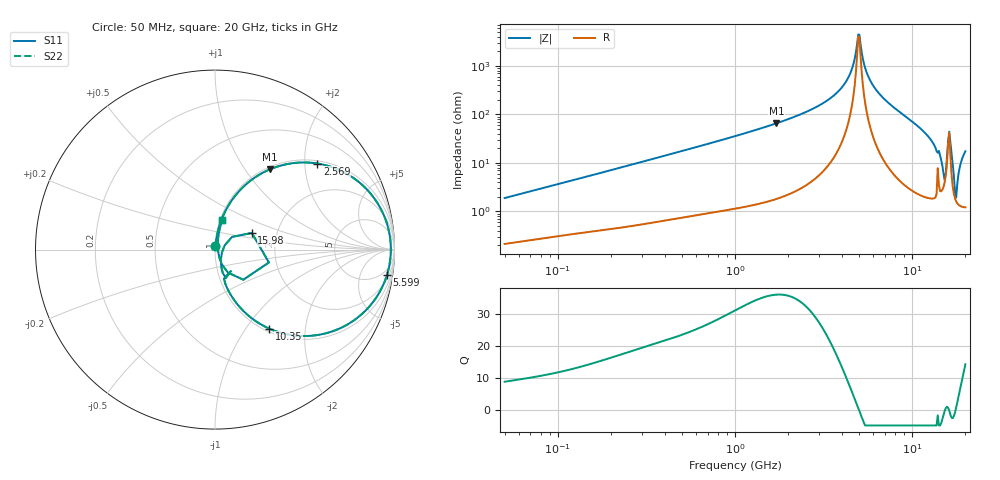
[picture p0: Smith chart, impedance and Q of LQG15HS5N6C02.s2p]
!Murata Part Number: LQG15HS5N6C02
!These Parameters are Measured in Series Mode Connection
!  o--[Z]--o
!Port1  Port2
!  o-------o
!Freq. Start=50[MHz] Stop=20[GHz], 401[Steps]
# Hz S RI R 50
!Freq.(Hz) S11(Real) S11(Imag) S21(Real) S21(Imag) S12(Real) S12(Imag) S22(Real) S22(Imag)
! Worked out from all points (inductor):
!   401 points, 50 MHz to 20 GHz, reference 50 ohm
!   read as one part in series: L = 5.91 nH near 51.52 MHz
!   highest Q = 36.2 at 1.715 GHz (marker M1), where L = 6.08 nH
!   self-resonance near 4.967 GHz
!   S11 on the Smith chart (normalised r, x): 50 MHz: 1.00, +0.04; 2.569 GHz: 1.07, +2.32; 5.599 GHz: 3, -13; 10.35 GHz: 1.05, -1.29; 15.98 GHz: 1.48, +0.29; 20 GHz: 1.02, +0.35
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5e7  0.00249 0.0187  0.9975 -0.0187  0.9975 -0.0187  0.00249 0.0187
1.364002e8  0.00598 0.0486  0.994 -0.0486  0.994 -0.0486  0.00598 0.0486
3.721004e8  0.0227 0.127  0.9773 -0.127  0.9773 -0.127  0.0227 0.127
1e9  0.1201 0.3094  0.8799 -0.3094  0.8799 -0.3094  0.1201 0.3094
1.714689e9  0.3053 0.4469  0.6947 -0.4469  0.6947 -0.4469  0.3053 0.4469
2.569357e9  0.5709 0.4795  0.4291 -0.4795  0.4291 -0.4795  0.5709 0.4795
2.728004e9  0.6189 0.4695  0.3811 -0.4695  0.3811 -0.4695  0.6189 0.4695
4.149438e9  0.93 0.215  0.07 -0.215  0.07 -0.215  0.93 0.215
4.539627e9  0.9658 0.1171  0.0342 -0.1171  0.0342 -0.1171  0.9658 0.1171
4.966507e9  0.9797 0.00897  0.0203 -0.00897  0.0203 -0.00897  0.9797 0.00897
5.117541e9  0.9789 -0.0284  0.0211 0.0284  0.0211 0.0284  0.9789 -0.0284
5.598765e9  0.9584 -0.1407  0.0416 0.1407  0.0416 0.1407  0.9584 -0.1407
7.442007e9  0.7244 -0.4247  0.2756 0.4247  0.2756 0.4247  0.7244 -0.4247
1.034674e10  0.3014 -0.4401  0.6986 0.4401  0.6986 0.4401  0.3014 -0.4401
1.295331e10  0.0857 -0.2486  0.9143 0.2486  0.9143 0.2486  0.0857 -0.2486
1.504638e10  0.0335 -0.0495  0.9665 0.0495  0.9665 0.0495  0.0335 -0.0495
1.550395e10  0.0536 0.0232  0.9464 -0.0232  0.9464 -0.0232  0.0536 0.0232
1.597544e10  0.205 0.0929  0.795 -0.0929  0.795 -0.0929  0.205 0.0929
1.646126e10  0.1576 -0.1678  0.8424 0.1678  0.8424 0.1678  0.1576 -0.1678
1.721783e10  0.0248 -0.0463  0.9752 0.0463  0.9752 0.0463  0.0248 -0.0463
1.774144e10  0.016 0.0102  0.984 -0.0102  0.984 -0.0102  0.016 0.0102
2e10  0.0402 0.1644  0.9598 -0.1644  0.9598 -0.1644  0.0402 0.1644
